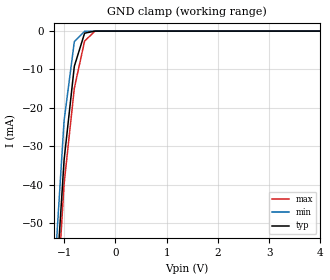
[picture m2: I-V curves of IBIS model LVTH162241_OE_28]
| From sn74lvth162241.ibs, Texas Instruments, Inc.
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|   Model LVTH162241 Input_OE_28
[Model]   LVTH162241_OE_28
Model_type  Input
Polarity   Non-Inverting
Vinl = 0.8V
Vinh = 2.0V
| variable   typ   min   max
C_comp   4pf   NA   NA
[Temperature Range]   40   -25   100
| Ambient temperature   25   -40   85
[Voltage range]   2.8   2.7   2.9
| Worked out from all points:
|   GND clamp passes 1 mA (typ) near -0.61 V on its own axis
[GND Clamp]
|   Voltage   I(typ)   I(min)   I(max)
-5V       -1.568A    -1.701A    -1.424A
-1.2V     -75.66mA   -65.99mA   -83.76mA
-1V       -33.63mA   -23.37mA   -39.86mA
-800mV    -9.157mA   -2.732mA   -14.86mA
-600mV    -552.4uA   -49.93uA   -2.615mA
-400mV    -1.257uA   -446.2nA   -49.82uA
5V        -36.12pA   86.59nA    -22.5pA
